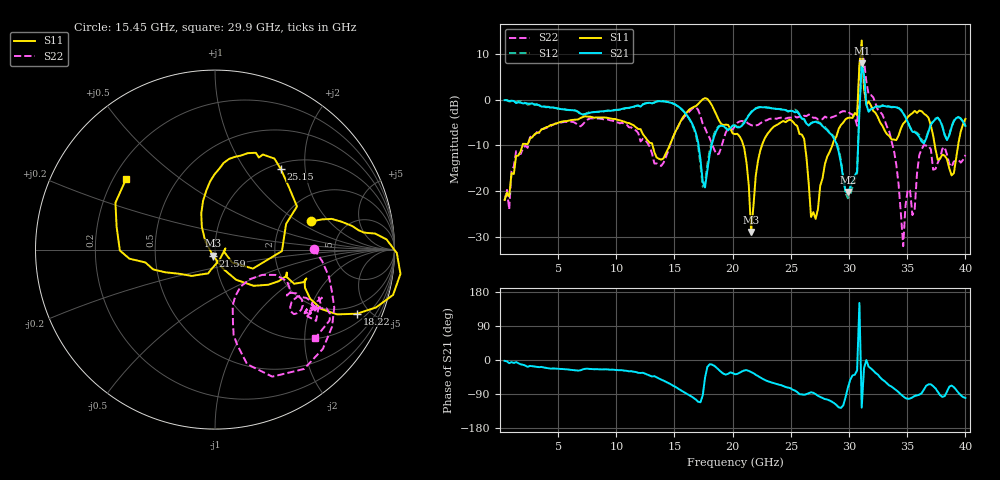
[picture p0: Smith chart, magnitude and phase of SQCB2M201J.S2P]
! Network Analyzer HP8722ES.07.66: Jul 25, 2000 Serial No. US39175408
! 27 Oct 2004  13:24:46
! Frequency  S11  S21  S12  S22
# HZ  S  DB R  50
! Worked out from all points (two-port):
!   201 points, 400 MHz to 40 GHz, reference 50 ohm
!   highest |S21| = 8.00 dB at 31.09 GHz (marker M1); lowest = -20.2 dB at 29.9 GHz (marker M2)
!   |S21| within 3 dB of the highest: 31.03 GHz to 31.3 GHz (262.7 MHz wide, 0.843 % of centre)
!   lowest |S11| = -29.0 dB at 21.59 GHz (marker M3), VSWR 1.07, Z = 48.9 - j3.34 ohm
!   |S11| at or under -10 dB: start of sweep to 1.941 GHz; 26.21 GHz to 28.56 GHz (2.349 GHz wide, 8.58 % of centre); 37.37 GHz to 39.38 GHz (2.002 GHz wide, 5.22 % of centre)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
!   |S22| runs from -32.1 to 10.3 dB; largest |S21 - S12| = 0.17
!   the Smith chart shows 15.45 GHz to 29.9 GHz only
!   S11 on the Smith chart (normalised r, x): 15.45 GHz: 2.85, +1.29; 18.22 GHz: 1.44, -4.17; 21.59 GHz: 0.98, -0.07; 25.15 GHz: 1.10, +1.49; 29.9 GHz: 0.25, +0.33
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4e8  -21.96 -97.6  -0.09 -2.4  -0.02 -1.9  -22.11 -95.3
7.132e9  -3.78 -91.5  -3.24 -24.6  -3.29 -25.4  -5.38 -125.8
1.3666e10  -12.94 -44.3  -0.29 -49.0  -0.32 -49.1  -14.34 121.0
1.5448e10  -5.11 16.4  -1.68 -78.1  -1.72 -78.9  -5.20 0.6
1.822e10  -1.23 -24.3  -9.64 -12.1  -8.97 -12.6  -9.70 -72.5
2.02e10  -7.54 -17.7  -5.65 -37.6  -5.59 -38.3  -5.76 -28.2
2.1586e10  -28.98 -106.6  -2.79 -31.8  -2.66 -33.1  -5.54 -37.6
2.2576e10  -9.56 98.3  -1.64 -49.7  -1.59 -51.1  -4.79 -27.9
2.515e10  -4.74 50.7  -2.45 -78.4  -2.37 -79.3  -3.93 -34.7
2.6932e10  -24.67 6.9  -4.91 -86.6  -4.82 -88.4  -3.97 -35.8
2.9902e10  -3.97 141.3  -20.24 -73.2  -21.61 -82.4  -2.56 -41.4
3.0694e10  -3.37 78.0  -15.75 -27.3  -16.21 -23.9  -5.69 -51.1
3.0892e10  7.73 31.7  -2.65 150.6  -1.76 150.1  6.88 -31.3
3.109e10  13.02 -46.5  8.00 -125.6  7.55 -123.0  10.28 131.4
3.1288e10  2.44 -48.3  5.29 -21.0  5.18 -18.5  8.62 -98.8
3.1486e10  -1.09 -71.5  -1.04 -0.1  -1.02 -0.0  3.97 -65.6
3.1684e10  -0.35 -88.8  -2.62 -17.4  -2.44 -18.1  1.17 -71.4
3.3466e10  -7.96 -126.9  -1.54 -67.4  -1.42 -66.4  -7.04 -115.8
3.4654e10  -5.23 -97.3  -2.95 -95.6  -2.85 -95.8  -32.12 -12.2
3.6832e10  -3.97 -154.6  -6.97 -64.3  -6.83 -65.5  -10.10 -17.3
3.8812e10  -16.58 158.5  -6.01 -67.4  -5.81 -69.3  -14.71 -31.2
4e10  -4.20 -1.6  -5.72 -100.4  -5.79 -100.8  -12.11 -64.1
